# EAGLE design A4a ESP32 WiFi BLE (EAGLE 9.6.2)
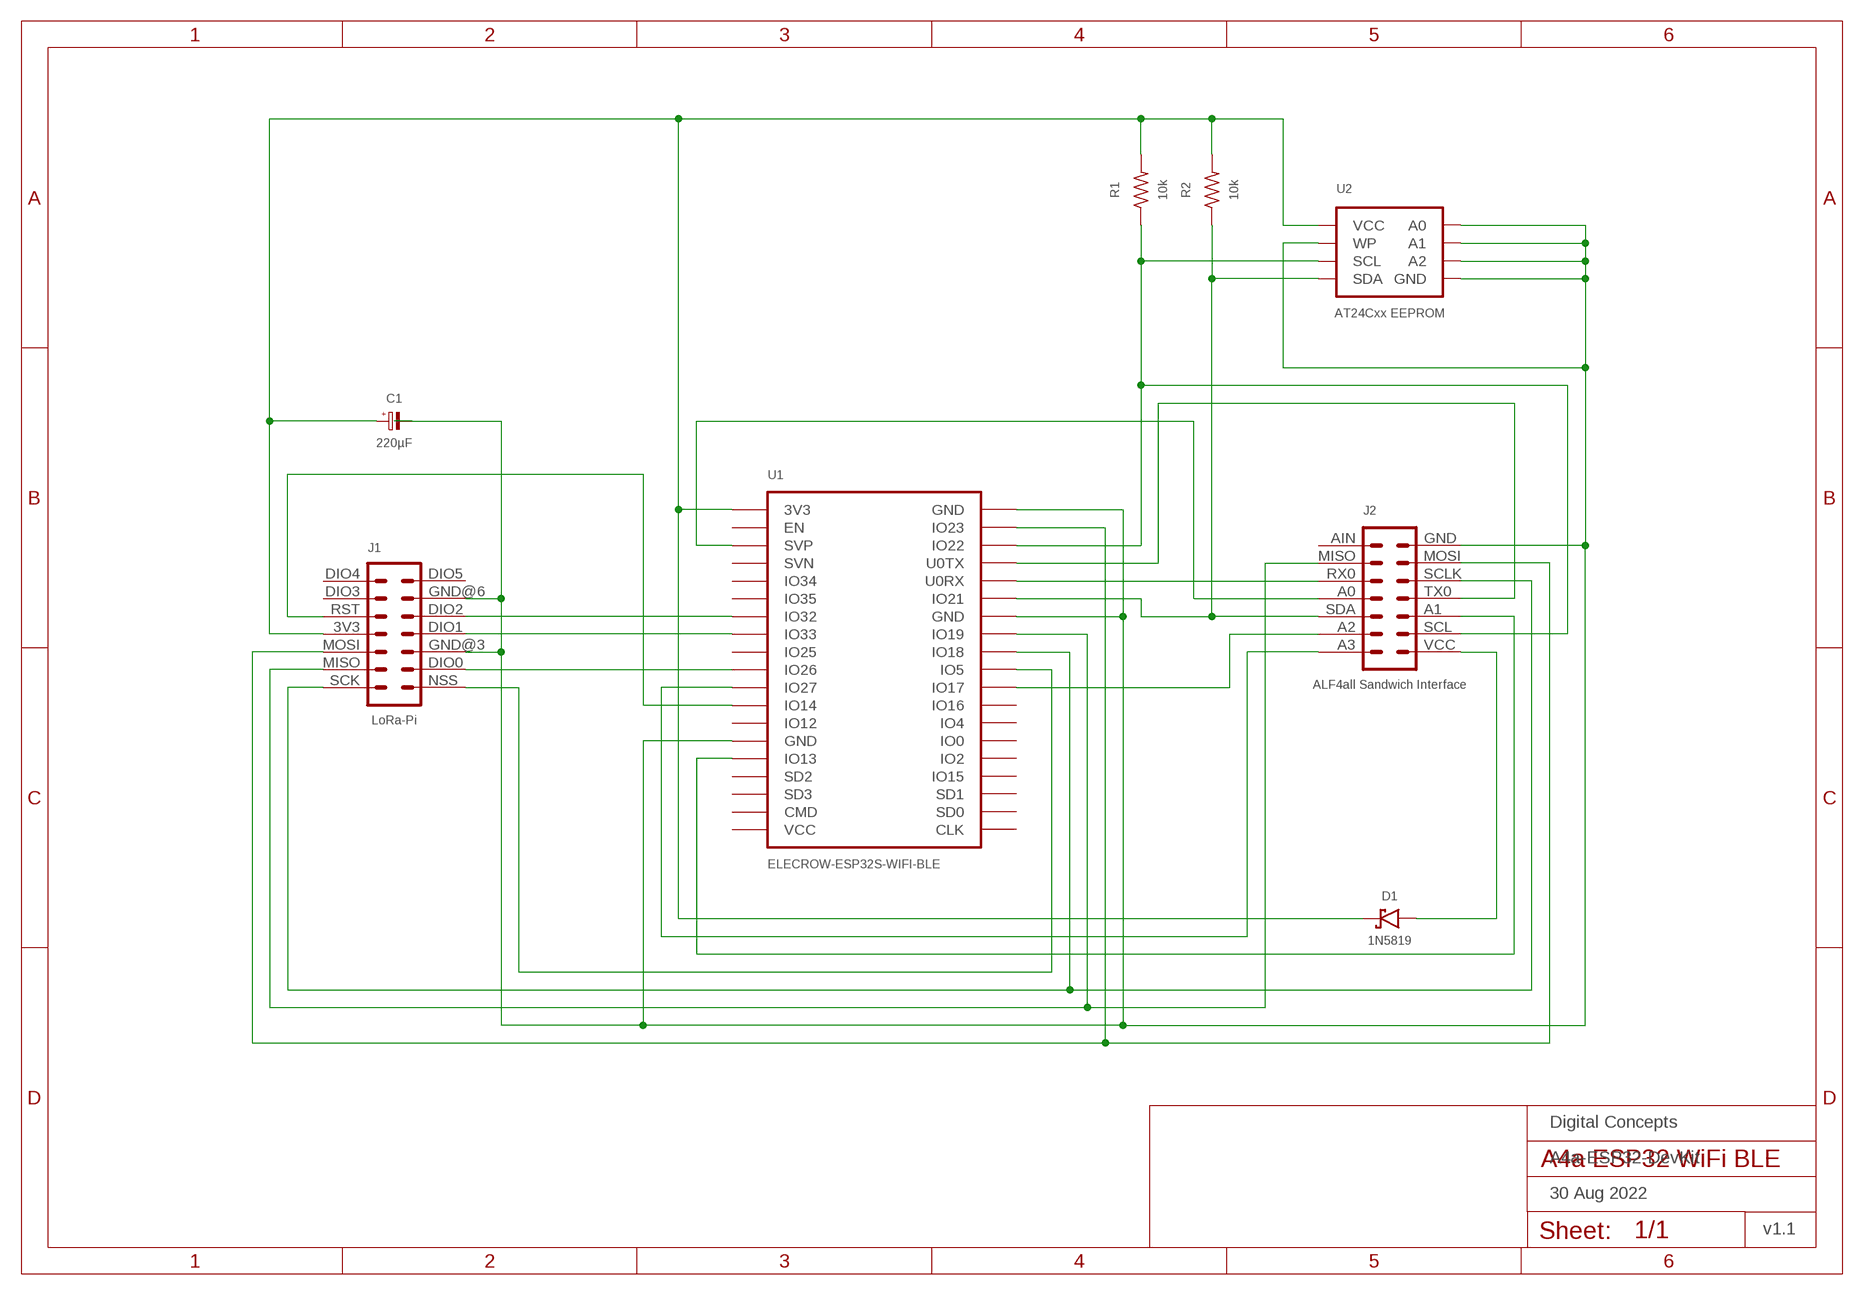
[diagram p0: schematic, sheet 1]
FRAME1 (A4L-LOC): DATE: 30 Aug 2022; OWNER: Digital Concepts; TITLE: A4a-ESP32-DevKit; VERSION: v1.1

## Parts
C1  220µF  CAPACITOR-3528-TANTALUM  [C3528-21]
D1  1N5819  DIODE-SCHOTTKY-1N5819  [SOD-123]
J1  LoRa-Pi  RFM95W-PI-HEADER  [RFM95W-PI]
J2  ALF4all Sandwich Interface  HEADER-2X7-ALF4ALL-PROCESSOR-B  [CONN_2X7-ALF4ALL-PROCESSOR-B]
R1  10k  RESISTORR0805  [R0805]
R2  10k  RESISTORR0805  [R0805]
U1  ELECROW-ESP32S-WIFI-BLE  [ELECROW-ESP32S-WIFI-BLE]
U2  AT24Cxx EEPROM  AT24CXX-EEPROM  [SOP-8]

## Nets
GND: C1.2(-) J1.GND@3 J1.GND@6 J2.GND U1.GND@13(GND) U1.GND@19(GND) U1.GND@33(GND) U2.P$1(A0) U2.P$2(A1) U2.P$3(A2) U2.P$4(GND) U2.P$7(WP)
N$2: J2.A3 U1.IO27
N$3: J2.A1 U1.IO13
N$4: J1.RST U1.IO14
N$5: D1.A J2.VCC
N$6: J1.SCK J2.SCLK U1.IO18
N$7: J2.RX0 U1.U0RX
N$9: J1.DIO0 U1.IO26
N$10: J2.SDA R2.1 U1.IO21 U2.P$5(SDA)
N$11: J2.SCL R1.1 U1.IO22 U2.P$6(SCL)
N$12: J1.MISO J2.MISO U1.IO19
N$13: J1.MOSI J2.MOSI U1.IO23
N$14: J2.TX0 U1.U0TX
N$15: J1.NSS U1.IO5
N$17: J2.A2 U1.IO17
N$21: J1.DIO1 U1.IO33
N$22: J1.DIO2 U1.IO32
N$23: J2.A0 U1.SVP
VCC: C1.1(+) D1.C J1.3V3 R1.2 R2.2 U1.3V3 U2.P$8(VCC)
Unconnected: J1.DIO3 J1.DIO4 J1.DIO5 J2.AIN U1.CLK U1.CMD U1.EN U1.IO0 U1.IO2 U1.IO4 U1.IO12 U1.IO15 U1.IO16 U1.IO25 U1.IO34 U1.IO35 U1.SD0 U1.SD1 U1.SD2 U1.SD3 U1.SVN U1.VCC

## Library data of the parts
C1 = digitalconcepts:CAPACITOR-3528-TANTALUM: Capacitor Tantalum 3528 (KEMET B)
D1 = digitalconcepts:DIODE-SCHOTTKY-1N5819: 1N5819 Schottky Diode SOD-123
J1 = digitalconcepts:RFM95W-PI-HEADER: RFM95W LoRa Wireless Transceiver Raspberry Pi Daughter Board
J2 = digitalconcepts:HEADER-2X7-ALF4ALL-PROCESSOR-B: ALF4all 'Sandwich' Processor (Bottom) 2x7 Pin Header Header soldered to underside of PCB
R1 R2 = digitalconcepts:RESISTOR: Resistor; SPICEPREFIX: R
U1 = digitalconcepts:ELECROW-ESP32S-WIFI-BLE: Elecrow ESP32S WiFi/BLE DevKit
U2 = digitalconcepts:AT24CXX-EEPROM: AT24Cxx EEPROM SOP-8

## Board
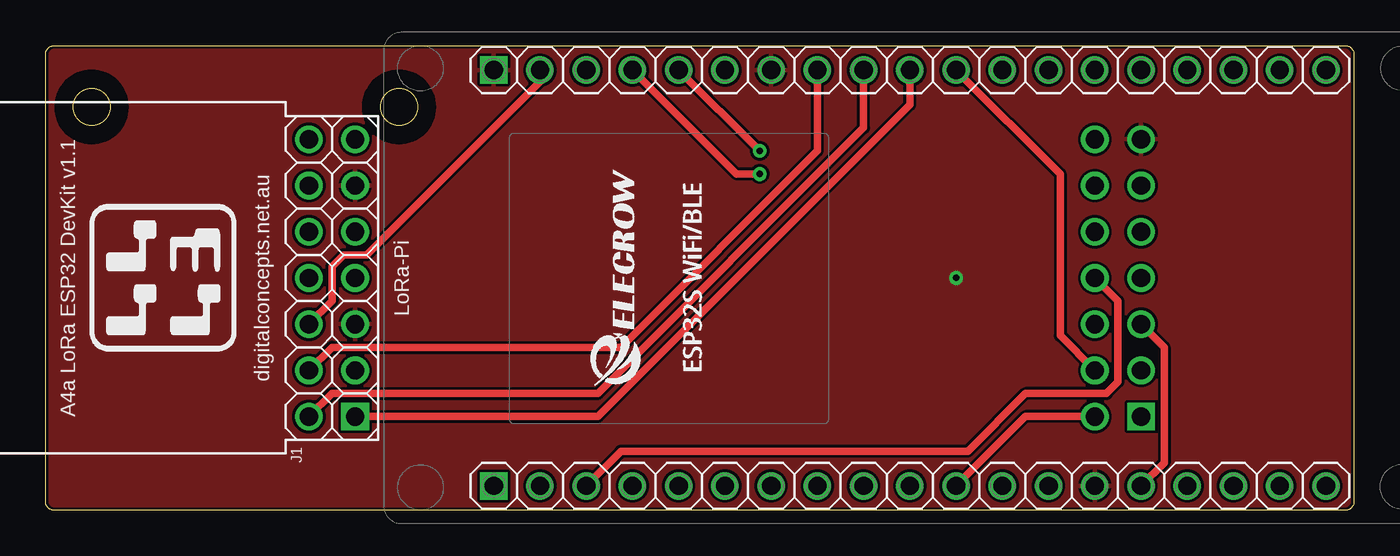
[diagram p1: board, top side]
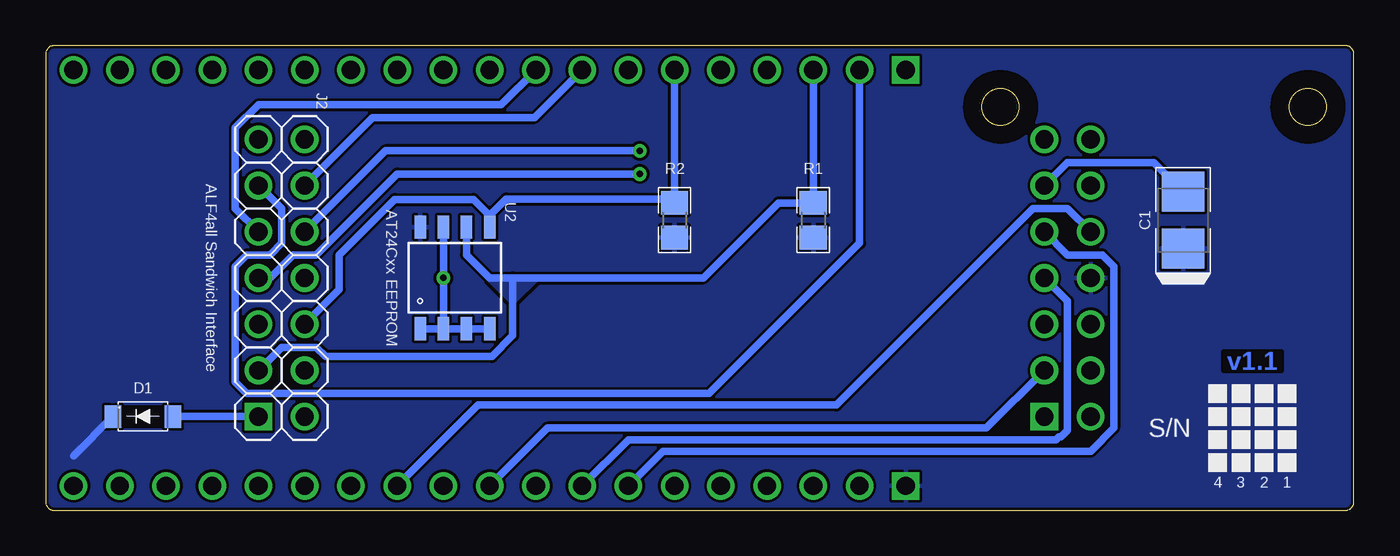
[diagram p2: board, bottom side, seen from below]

Size 71.89 x 25.56 mm. Coordinates in mm from the lower left corner, seen from the top.
Outline: 87 segments
Outline: circle at 19.42,22.18 radius 1.02
Outline: circle at 2.53,22.18 radius 1.02
Copper layers (1*16): Top 0.035mm / dielectric 1.5mm / Bottom 0.035mm
Design rules "default *": minimum track width 6mil, minimum drill 0.35mm, track to track 6mil, track to pad 6mil, pad to pad 6mil, via to via 6mil, smd to smd 6mil, copper to edge 6mil, drill to drill 6mil, minimum pad ring 10mil, minimum via ring 8mil, stop-mask expansion 4mil, vias tented up to drill 0mil, thermal gap 6mil

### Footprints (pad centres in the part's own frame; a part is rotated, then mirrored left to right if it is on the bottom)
C3528-21 = smd 2.21 x 2.35: 1 -1.565,0; 2 1.565,0
SOD-123 = smd 0.91 x 1.22: A -1.65,0; C 1.65,0
RFM95W-PI = drill 1 pad 1.524: 3V3 7.62,2.54; DIO0 2.54,0; DIO1 7.62,0; DIO2 10.16,0; DIO3 12.7,2.54; DIO4 15.24,2.54; DIO5 15.24,0; GND@3 5.08,0; GND@6 12.7,0; MISO 2.54,2.54; MOSI 5.08,2.54; RST 10.16,2.54; SCK 0,2.54 | drill 1 pad 1.524 square: NSS 0,0
CONN_2X7-ALF4ALL-PROCESSOR-B = drill 1 pad 1.524: A0 7.62,2.54; A1 5.08,0; A2 2.54,2.54; A3 0,2.54; AIN 15.24,2.54; GND 15.24,0; MISO 12.7,2.54; MOSI 12.7,0; RX0 10.16,2.54; SCL 2.54,0; SCLK 10.16,0; SDA 5.08,2.54; TX0 7.62,0 | drill 1 pad 1.524 square: VCC 0,0
R0805 = smd 1.3 x 1.5: 1 -0.95,0; 2 0.95,0
ELECROW-ESP32S-WIFI-BLE = drill 1 square: 3V3 -22.86,45.72; GND@19 0,45.72 | drill 1: CLK 0,0; CMD -22.86,2.54; EN -22.86,43.18; GND@13 0,30.48; GND@33 -22.86,12.7; IO0 0,12.7; IO2 0,10.16; IO4 0,15.24; IO5 0,22.86; IO12 -22.86,15.24; IO13 -22.86,10.16; IO14 -22.86,17.78; IO15 0,7.62; IO16 0,17.78; IO17 0,20.32; IO18 0,25.4; IO19 0,27.94; IO21 0,33.02; IO22 0,40.64; IO23 0,43.18; IO25 -22.86,25.4; IO26 -22.86,22.86; IO27 -22.86,20.32; IO32 -22.86,30.48; IO33 -22.86,27.94; IO34 -22.86,35.56; IO35 -22.86,33.02; SD0 0,2.54; SD1 0,5.08; SD2 -22.86,7.62; SD3 -22.86,5.08; SVN -22.86,38.1; SVP -22.86,40.64; U0RX 0,35.56; U0TX 0,38.1; VCC -22.86,0
SOP-8 = smd 0.635 x 1.27: P$1 -1.905,-2.794; P$2 -0.635,-2.794; P$3 0.635,-2.794; P$4 1.905,-2.794; P$5 1.905,2.794; P$6 0.635,2.794; P$7 -0.635,2.794; P$8 -1.905,2.794

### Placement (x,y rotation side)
C1  9.39,15.96 90 bottom
D1  66.54,5.16 180 bottom
J1  17.01,5.16 90 top
J2  60.19,5.16 90 top
R1  29.71,15.96 270 bottom
R2  37.33,15.96 270 bottom
U1  70.35,24.21 90 top
U2  49.39,12.78 0 bottom

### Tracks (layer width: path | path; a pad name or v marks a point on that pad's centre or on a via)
$X1
  cutout Top: 2.53,24.21 arc180 2.53,20.15 arc180
$X2
  cutout Bottom: 2.53,24.21 arc180 2.53,20.15 arc180
$X3
  cutout Top: 19.42,24.21 arc180 19.42,20.15 arc180
$X4
  cutout Bottom: 19.42,24.21 arc180 19.42,20.15 arc180
GND  (via drill 0.35)
  Bottom 0.406: U2.P$1 U2.P$2 | U2.P$7 v50.03,12.78 U2.P$2 | U2.P$2 U2.P$3 U2.P$4 | J1.GND@6 15.74,19.13 11,19.13 C1.2
  pour Top (rank 5): -1.41,26.75 72.89,26.75 72.89,-1.19 -1.41,-1.19
N$2
  Top 0.406: U1.IO27 53.84,5.16 J2.A3
N$3
  Top 0.406: U1.IO13 61.46,2.62 61.46,8.97 J2.A1
N$4
  Bottom 0.406: J1.RST 15.74,16.59 17.64,16.59 28.44,5.8 48.12,5.8 U1.IO14
N$5
  Bottom 0.406: J2.VCC D1.A
N$6
  Top 0.406: J1.SCK 15.74,6.43 30.34,6.43 44.95,21.04 U1.IO18
  Bottom 0.406: J2.SCLK 61.46,16.59 61.46,21.04 60.19,22.31 46.85,22.31 U1.IO18
N$7  (via drill 0.35)
  Top 0.406: U1.U0RX v39.23,19.77
  Bottom 0.406: J2.RX0 53.2,19.77 v39.23,19.77
N$9
  Bottom 0.406: J1.DIO0 20.18,4.53 44.31,4.53 U1.IO26
N$10
  Bottom 0.406: U2.P$5 47.49,16.21 | 47.49,16.21 48.38,17.1 52.7,17.1 55.74,14.05 55.74,12.15 J2.SDA | 47.49,16.21 46.57,17.13 37.55,17.13 R2.1 U1.IO21
N$11
  Bottom 0.406: J2.SCL 58.92,8.97 57.01,8.97 56.51,8.46 47.36,8.46 46.22,9.61 46.22,12.78 | U2.P$6 48.76,14.05 47.49,12.78 46.22,12.78 | 46.22,12.78 35.74,12.78 31.62,16.91 R1.1 U1.IO22
  pour Bottom: 47.49,12.78 44.95,12.78 46.22,11.51
N$12
  Top 0.406: J1.MISO 15.74,8.97 31.61,8.97 42.41,19.77 U1.IO19
  Bottom 0.406: J2.MISO 53.91,21.6 45.02,21.6 U1.IO19
N$13
  Top 0.406: J1.MOSI 15.74,11.51 15.74,13.42 16.37,14.05 17.64,14.05 27.17,23.58 U1.IO23
  Bottom 0.406: J2.MOSI 58.92,16.59 58.92,14.69 59.55,14.05 60.82,14.05 61.46,13.42 61.46,7.07 60.82,6.43 35.42,6.43 27.17,14.69 U1.IO23
N$14  (via drill 0.35)
  Top 0.406: v39.23,18.5 37.96,18.5 U1.U0TX
  Bottom 0.406: J2.TX0 59.55,12.78 58.28,14.05 57.01,14.05 52.57,18.5 v39.23,18.5
N$15
  Top 0.406: U1.IO5 47.49,22.31 30.34,5.16 J1.NSS
N$17
  Top 0.406: J2.A2 55.74,9.61 55.74,18.5 U1.IO17
N$21
  Bottom 0.406: J1.DIO1 15.74,11.51 15.74,4.41 16.1,4.04 16.22,4.04 16.37,3.89 39.87,3.89 U1.IO33
N$22
  Bottom 0.406: J1.DIO2 15.74,14.05 13.83,14.05 13.2,13.42 13.2,4.53 14.47,3.26 37.96,3.26 U1.IO32
N$23
  Top 0.406: J2.A0 58.92,11.51 58.92,7.07 58.28,6.43 53.84,6.43 50.66,3.26 31.61,3.26 U1.SVP
VCC
  Bottom 0.406: D1.C 70.35,3
  pour Bottom (rank 5): -0.77,26.12 72.25,26.12 72.25,-0.55 -0.77,-0.55

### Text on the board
Bottom: v1.1
tPlace: A4a LoRa ESP32 DevKit v1.1 | digitalconcepts.net.au
bPlace: S/N | 1 | 2 | 3 | 4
